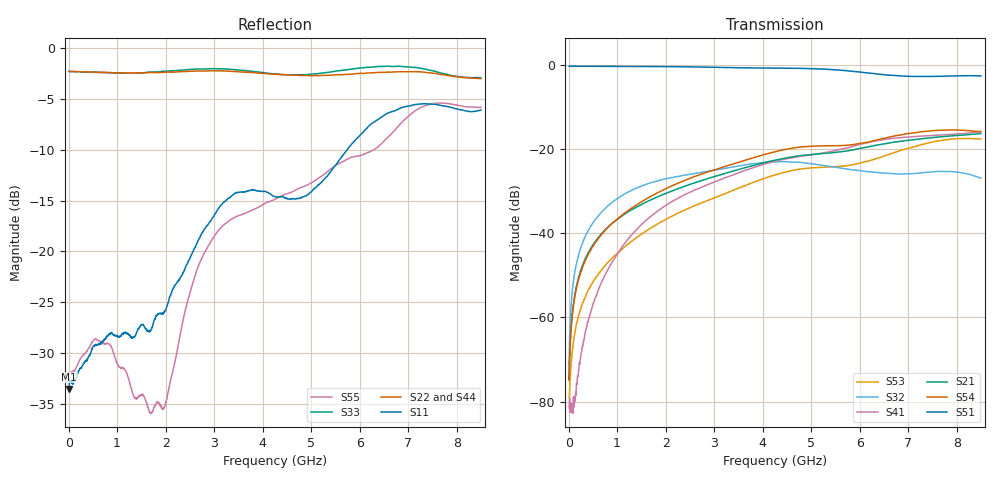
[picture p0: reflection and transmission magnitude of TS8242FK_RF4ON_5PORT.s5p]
! Created with skrf (http://scikit-rf.org).
# Hz S RI R 50.0
!freq ReS11 ImS11 ReS12 ImS12 ReS13 ImS13
! ReS14 ImS14 ReS15 ImS15
! ReS21 ImS21 ReS22 ImS22 ReS23 ImS23
! ReS24 ImS24 ReS25 ImS25
! ReS31 ImS31 ReS32 ImS32 ReS33 ImS33
! ReS34 ImS34 ReS35 ImS35
! ReS41 ImS41 ReS42 ImS42 ReS43 ImS43
! ReS44 ImS44 ReS45 ImS45
! ReS51 ImS51 ReS52 ImS52 ReS53 ImS53
! ReS54 ImS54 ReS55 ImS55
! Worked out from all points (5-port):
!   1601 points, 10 MHz to 8.5 GHz, reference 50 ohm
!   strongest paths, dB at 10 MHz, 2.132 GHz, 4.255 GHz, 6.378 GHz, 8.5 GHz:
!     S51: -0.3, -0.4, -0.7, -2.1, -2.6
!     S54: -75.0, -28.7, -20.6, -17.7, -15.8
!     S21: -74.7, -29.9, -22.6, -19.0, -16.3
!     S41: -81.5, -32.4, -22.9, -17.9, -15.8
!     S32: -71.1, -26.7, -23.0, -25.5, -26.9
!     S53: -79.0, -35.9, -26.1, -22.1, -17.6
!   lowest |S11| = -33.6 dB at 10 MHz (marker M1), VSWR 1.04, Z = 52.1 + j0.362 ohm
!   |S11| at or under -10 dB: start of sweep to 5.744 GHz
